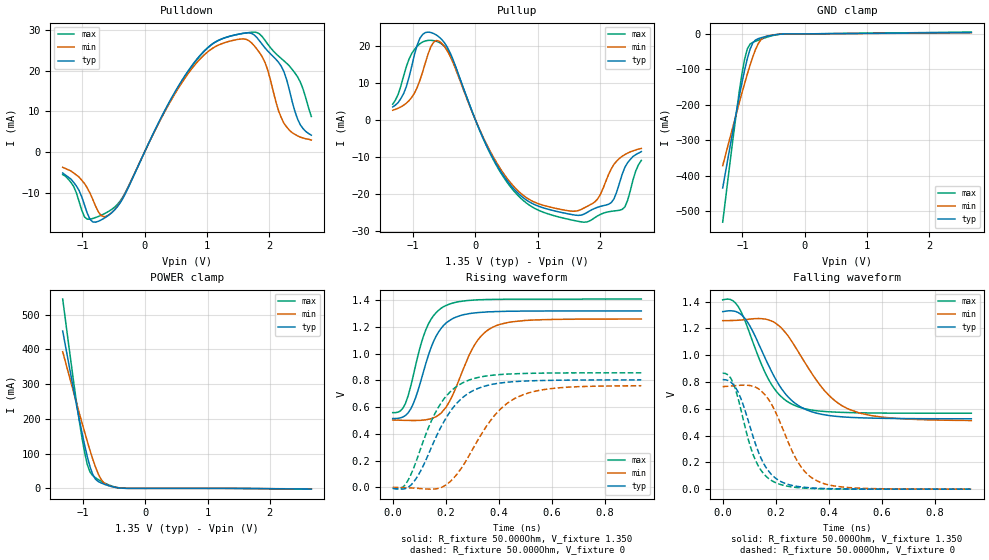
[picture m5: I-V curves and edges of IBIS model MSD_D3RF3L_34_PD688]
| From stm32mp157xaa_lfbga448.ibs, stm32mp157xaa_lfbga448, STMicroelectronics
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[Model] MSD_D3RF3L_34_PD688
Model_type   I/O
C_comp 2.452pF   2.367pF   2.576pF
Vinh = 810.000mV
Vinl = 540.000mV
Vmeas = 675.000mV
Vref = 675.000mV
[Model Spec]
Vinh   810.000mV   777.000mV   860.000mV
Vinl   540.000mV   507.000mV   590.000mV
Vmeas   675.000mV   642.000mV   725.000mV
Vref   675.000mV   642.000mV   725.000mV
[Temperature Range]   25.000   125.000   -40.000
[Voltage Range]   1.350V   1.283V   1.450V
[GND Clamp Reference]   0.00V   0.00V   0.00V
[Pulldown Reference]   0.00V   0.00V   0.00V
[POWER Clamp Reference]   1.350V   1.283V   1.450V
[Pullup Reference]   1.350V   1.283V   1.450V
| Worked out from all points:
|   slope of the pulldown table from 0 to 0.203 V, typ, clamps not added: 31 ohm
|   slope of the pullup table from 0 to 0.203 V, typ, clamps not added: 26.2 ohm
|   GND clamp passes 1 mA (typ) near -0.40 V on its own axis
|   POWER clamp passes 1 mA (typ) near -0.41 V on its own axis
|   rising waveform, R_fixture 50.000Ohm, V_fixture 1.350: 20-80 % time 84.6ps typ, 106ps min, 75.1ps max; typ from 0.515 V to 1.32 V
|   rising waveform, R_fixture 50.000Ohm, V_fixture 0: 20-80 % time 134ps typ, 158ps min, 119ps max; typ from -0.006 V to 0.804 V
|   falling waveform, R_fixture 50.000Ohm, V_fixture 1.350: 20-80 % time 132ps typ, 164ps min, 113ps max; typ from 1.32 V to 0.525 V
|   falling waveform, R_fixture 50.000Ohm, V_fixture 0: 20-80 % time 90.2ps typ, 111ps min, 78.6ps max; typ from 0.818 V to 0 V
[GND Clamp]
-1.318V   -434mA     -371.3mA   -530.2mA
-1.142V   -261.5mA   -253.5mA   -281.3mA
-1.055V   -179mA     -196mA     -166.2mA
-1.011V   -139.8mA   -167.8mA   -115.1mA
-966.7mV  -103mA     -140.4mA   -72.11mA
-922.7mV  -70.13mA   -113.7mA   -42.44mA
-878.8mV  -43.47mA   -88.39mA   -29mA
-790.9mV  -17.29mA   -44.25mA   -20.79mA
-703mV    -11.11mA   -16.27mA   -15.06mA
-527.3mV  -4.042mA   -3.425mA   -5.39mA
-307.6mV  -133.2uA   -195.4uA   -121.4uA
2.68V     3.865mA    3.009mA    5.016mA
[Power Clamp]
-1.33V    453.1mA    393.5mA    545.2mA
-1.111V   242.6mA    247.9mA    251.8mA
-1.023V   163mA      190.9mA    148.8mA
-978.8mV  125.7mA    162.9mA    104.3mA
-934.9mV  91.65mA    135.6mA    68.75mA
-890.9mV  62.25mA    109.3mA    47.1mA
-847mV    39.9mA     84.29mA    36.58mA
-803mV    26.52mA    61.46mA    30.46mA
-715.1mV  15.81mA    26.66mA    20.93mA
-671.2mV  12.58mA    16.56mA    16.75mA
-407.6mV  927uA      1.209mA    1.127mA
2.668V    -1.945mA   -1.621mA   -2.312mA
[Pulldown]
-1.318V   -5.2mA     -3.8mA     -5.6mA
-922.7mV  -15.11mA   -8.9mA     -16.55mA
-703mV    -16.78mA   -15.62mA   -15.62mA
-571.2mV  -15.5mA    -15.46mA   -14.56mA
-351.5mV  -11.48mA   -11.33mA   -11.11mA
747mV     20.95mA    20.23mA    20.78mA
1.098V    26.63mA    25.53mA    26.63mA
1.582V    29.15mA    27.78mA    29.12mA
1.933V    25.61mA    22.07mA    27.48mA
2.197V    21.04mA    8.4mA      22.95mA
2.461V    8mA        3.9mA      18.4mA
2.68V     4.1mA      2.9mA      8.7mA
[Pullup]
-1.33V    3.5mA      2.605mA    4.252mA
-1.155V   7.1mA      3.962mA    11.86mA
-978.8mV  17.8mA     7.282mA    19.11mA
-715.1mV  23.66mA    19.86mA    21.56mA
-451.5mV  19.67mA    18.67mA    18.99mA
251.5mV   -9.374mA   -8.925mA   -9.6mA
866.7mV   -22.21mA   -21.56mA   -23.09mA
1.702V    -25.8mA    -24.27mA   -27.63mA
1.965V    -23.67mA   -21.43mA   -26.01mA
2.185V    -22.4mA    -13.26mA   -24.77mA
2.361V    -14.7mA    -9.838mA   -24.24mA
2.668V    -8.6mA     -7.748mA   -10.98mA
[Ramp]
R_load=50.000Ohm
dV/dt_r   479.400mV/110.000ps  453.119mV/133.000ps  509.280mV/97.000ps
dV/dt_f   479.400mV/111.500ps  453.119mV/139.000ps  509.280mV/96.000ps
[Rising waveform]
R_fixture=50.000Ohm
V_fixture=1.350
V_fixture_min=1.283
V_fixture_max=1.450
0s        515.3mV    504.4mV    559.2mV
39ps      527mV      502mV      594.1mV
68ps      586.7mV    500.8mV    756.2mV
125ps     926.6mV    505.8mV    1.179V
163ps     1.128V     528.5mV    1.305V
202ps     1.23V      601.8mV    1.361V
307ps     1.304V     1.059V     1.401V
384ps     1.314V     1.204V     1.406V
537ps     1.318V     1.252V     1.407V
938ps     1.319V     1.259V     1.408V
[Rising waveform]
R_fixture=50.000Ohm
V_fixture=0
0s        -6.425mV   755.1uV    -5.776mV
39ps      -11.69mV   -719uV     3.316mV
77ps      36.08mV    -4.229mV   135.1mV
173ps     416.6mV    -5.985mV   601.7mV
221ps     579.3mV    51.31mV    722.9mV
269ps     680.3mV    175mV      787.1mV
384ps     773.9mV    538mV      840.5mV
489ps     794.5mV    690.8mV    851.5mV
642ps     801.9mV    747.1mV    856mV
938ps     804.2mV    760.3mV    856.8mV
[Falling waveform]
R_fixture=50.000Ohm
V_fixture=1.350
V_fixture_min=1.283
V_fixture_max=1.450
0s        1.325V     1.258V     1.413V
48ps      1.327V     1.26V      1.39V
87ps      1.266V     1.266V     1.242V
144ps     1.048V     1.273V     942mV
183ps     883.8mV    1.256V     785.1mV
269ps     647.2mV    1.077V     627.3mV
384ps     555.1mV    735.5mV    580mV
470ps     537.2mV    601.9mV    572mV
604ps     528.8mV    537.3mV    567.9mV
938ps     525.3mV    512.5mV    566.8mV
[Falling waveform]
R_fixture=50.000Ohm
V_fixture=0
0s        817.7mV    765.4mV    866.1mV
39ps      783.1mV    771.4mV    795.5mV
68ps      679.3mV    775.7mV    599.6mV
96ps      512.9mV    775.1mV    374.3mV
125ps     329.1mV    760.5mV    209.4mV
163ps     163mV      696.9mV    96.96mV
202ps     78.12mV    563.8mV    46.35mV
288ps     18.62mV    189.1mV    10.67mV
365ps     6.379mV    53.51mV    3.025mV
938ps     10.44uV    101uV      -2.578uV
